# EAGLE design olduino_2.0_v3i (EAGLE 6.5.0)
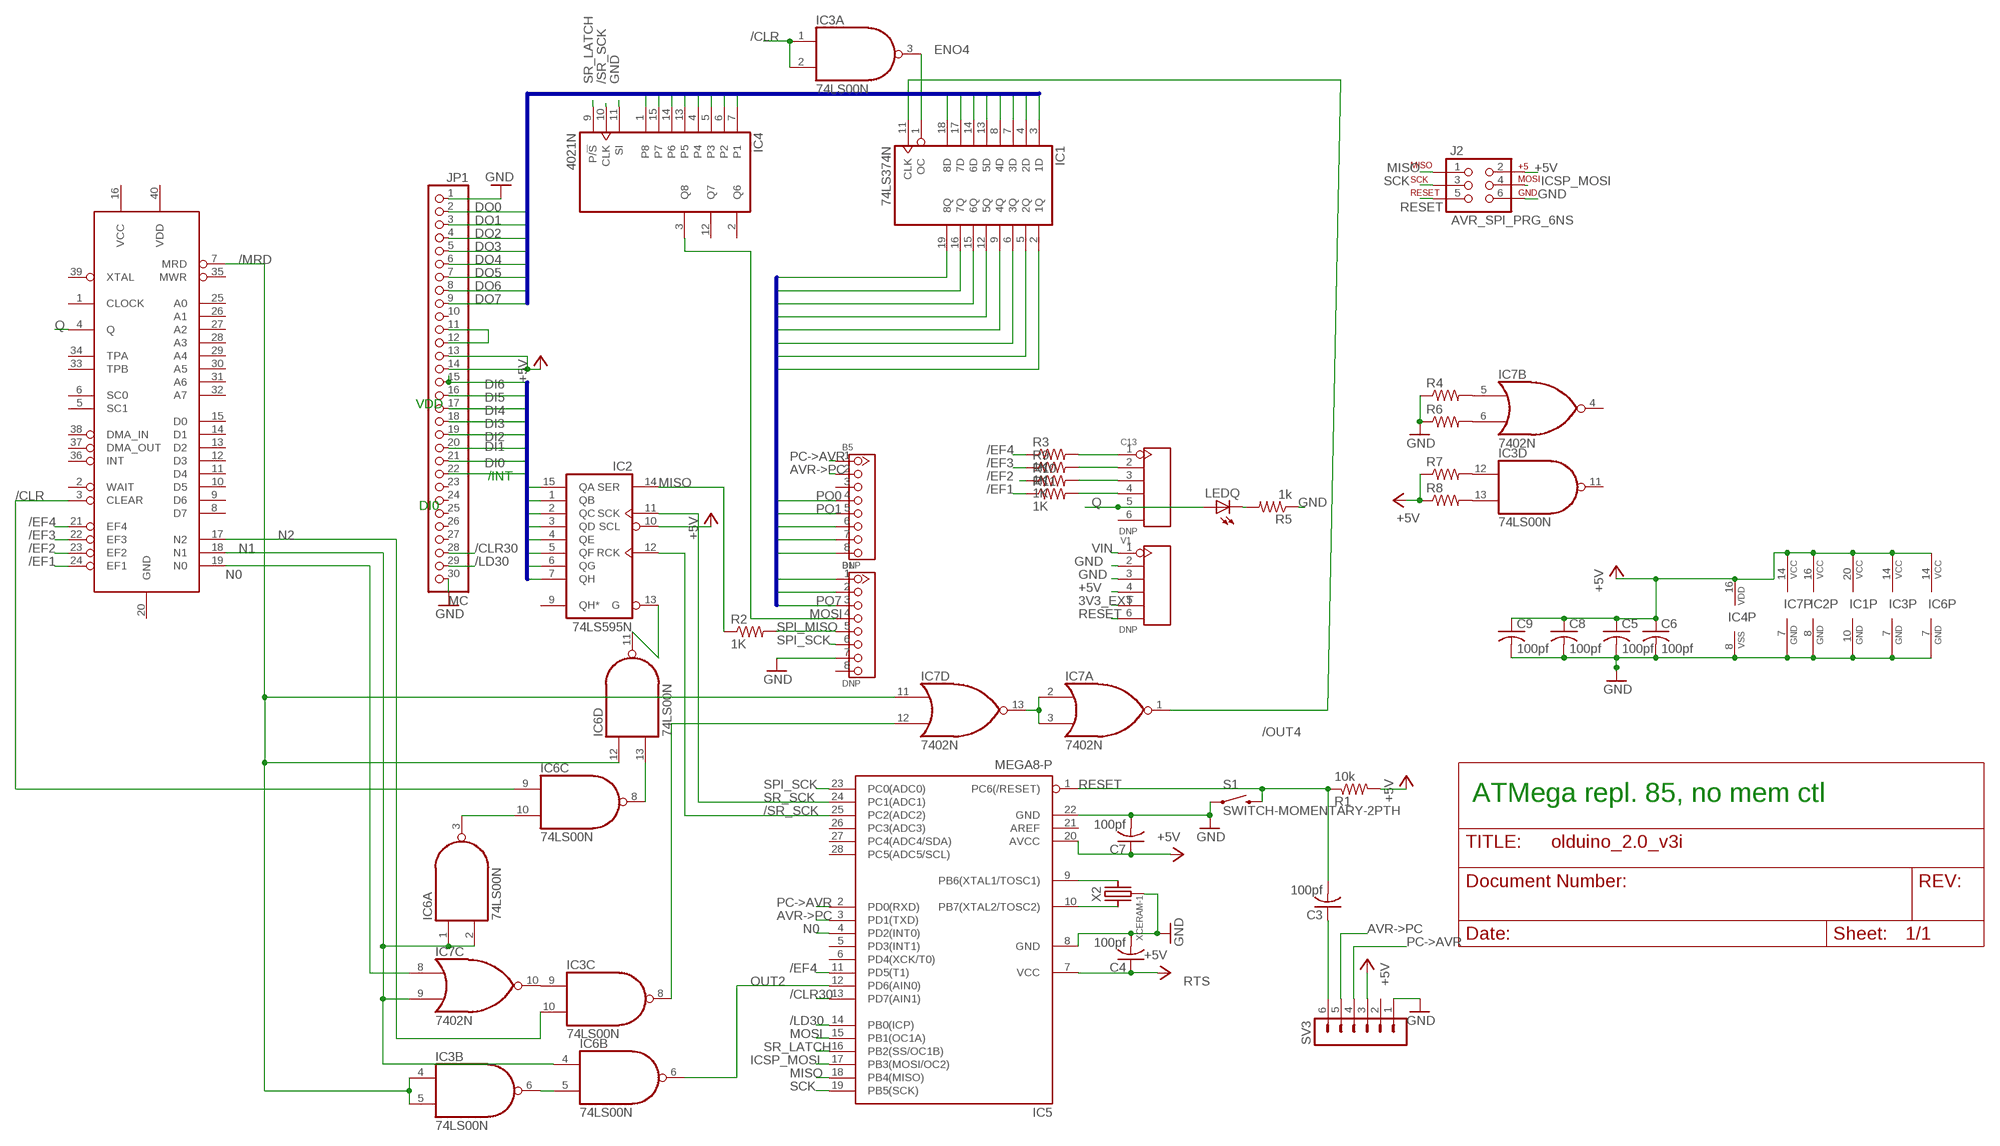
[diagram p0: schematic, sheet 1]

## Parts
B1  DNP  CK_1X8DD  [CK_1X8]
B5  DNP  CK_1X8DD  [CK_1X8]
C3  100pf  C-US025-025X050  [C025-025X050]
C4  100pf  C-US025-025X050  [C025-025X050]
C5  100pf  C-US025-025X050  [C025-025X050]
C6  100pf  C-US025-025X050  [C025-025X050]
C7  100pf  C-US025-025X050  [C025-025X050]
C8  100pf  C-US025-025X050  [C025-025X050]
C9  100pf  C-US025-025X050  [C025-025X050]
C13  DNP  CK_16  [CK_1*6]
IC1  74LS374N  [DIL20]
IC2  74LS595N  [DIL16]
IC3  74LS00N  [DIL14]
IC4  4021N  [DIL16]
IC5  MEGA8-P  [DIL28-3]
IC6  74LS00N  [DIL14]
IC7  7402N  [DIL14]
IC8  CDP1802BCE  CDP1802BCECDP1802BCE  [DIL40]
J2  AVR_SPI_PRG_6NS  [2X3-NS]
JP1  MC  PINHEAD_PINHD-1X30  [PINHEAD_1X30]
LEDQ  LED3MM  [LED3MM]
R1  10k  R-US_0204/2V  [0204V]
R2  1K  R-US_0204/2V  [0204V]
R3  1K  R-US_0204/2V  [0204V]
R4  R-US_0204/2V  [0204V]
R5  1k  R-US_0204/2V  [0204V]
R6  R-US_0204/2V  [0204V]
R7  R-US_0204/2V  [0204V]
R8  R-US_0204/2V  [0204V]
R9  1K  R-US_0204/2V  [0204V]
R10  1K  R-US_0204/2V  [0204V]
R11  1K  R-US_0204/2V  [0204V]
S1  SWITCH-MOMENTARY-2PTH  [TACTILE-PTH]
SV3  MA06-1  [MA06-1]
V1  DNP  CK_16  [CK_1*6]
X2  XCERAM-1  [XTAL-3]

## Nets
3V3_EXT: V1.5
+5V [power]: C4.1 C5.1 C6.1 C7.1 C8.1 C9.1 IC1.20(VCC) IC2.10(SCL) IC2.16(VCC) IC3.14(P:VCC) IC4.16(VDD) IC5.7(VCC) IC5.20(AVCC) IC6.14(P:VCC) IC7.14(P:VCC) J2.2 JP1.13 JP1.14 R1.2 R7.1 R8.1 SV3.3 V1.4
/CLR: IC3.1(A:I0) IC3.2(A:I1) IC6.9(C:I0) IC8.3(CLEAR)
/CLR30: IC5.13(PD7(AIN1)) JP1.28
/EF1: IC8.24(EF1) R11.1
/EF2: IC8.23(EF2) R10.1
/EF3: IC8.22(EF3) R9.1
/EF4: IC5.11(PD5(T1)) IC8.21(EF4) R3.1
/LD30: IC5.14(PB0(ICP)) JP1.29
/MRD: IC3.4(B:I0) IC3.5(B:I1) IC6.12(D:I0) IC7.11(D:I0) IC8.7(MRD)
/OUT4: IC1.11(CLK) IC7.1(A:O)
/SR_SCK: IC2.12(RCK) IC4.10(CLK) IC5.25(PC2(ADC2))
AVR->PC: B5.2 IC5.3(PD1(TXD)) SV3.5
DI0: IC2.15(QA) JP1.22
DI1: IC2.1(QB) JP1.21
DI2: IC2.2(QC) JP1.20
DI3: IC2.3(QD) JP1.19
DI4: IC2.4(QE) JP1.18
DI5: IC2.5(QF) JP1.17
DI6: IC2.6(QG) JP1.16
DI7: IC2.7(QH) JP1.15
DO0: IC1.3(1D) IC4.7(P1) JP1.2
DO1: IC1.4(2D) IC4.6(P2) JP1.3
DO2: IC1.7(3D) IC4.5(P3) JP1.4
DO3: IC1.8(4D) IC4.4 JP1.5
DO4: IC1.13(5D) IC4.13(P5) JP1.6
DO5: IC1.14(6D) IC4.14(P6) JP1.7
DO6: IC1.17(7D) IC4.15(P7) JP1.8
DO7: IC1.18(8D) IC4.1(P8) JP1.9
ENO4: IC1.1(OC) IC3.3(A:O)
GND [GND]: B1.7 C4.2 C5.2 C6.2 C7.2 C8.2 C9.2 IC1.10(GND) IC2.8(GND) IC3.7(P:GND) IC4.8(VSS) IC4.11(SI) IC5.8(GND) IC5.22(GND) IC6.7(P:GND) IC7.7(P:GND) J2.6 JP1.1 JP1.30 R4.1 R5.1 R6.1 S1.1 SV3.1 V1.2 V1.3 X2.P$2(GND)
ICSP_MOSI: IC5.17(PB3(MOSI/OC2)) J2.4
IO4: IC3.8(C:O) IC7.12(D:I1)
MISO: IC2.14(SER) IC5.18(PB4(MISO)) J2.1 R2.1
MOSI: B1.4 IC4.3(Q8) IC5.15(PB1(OC1A))
N0: IC5.4(PD2(INT0)) IC7.8(C:I0) IC8.19(N0)
N1: IC6.1(A:I0) IC6.2(A:I1) IC6.4(B:I0) IC7.9(C:I1) IC8.18(N1)
N2: IC3.10(C:I1) IC8.17(N2)
N$1: IC3.6(B:O) IC6.5(B:I1)
N$2: C13.1 R3.2
N$3: JP1.11 JP1.12
N$4: IC2.13(G) IC6.11(D:O)
N$5: IC7.2(A:I0) IC7.3(A:I1) IC7.13(D:O)
N$6: IC5.10(PB7(XTAL2/TOSC2)) X2.P$1
N$7: IC5.9(PB6(XTAL1/TOSC1)) X2.P$3
N$8: IC6.3(A:O) IC6.10(C:I1)
N$9: IC7.5(B:I0) R4.2
N$10: IC7.6(B:I1) R6.2
N$11: LEDQ.K(C) R5.2
N$12 [power]: IC3.12(D:I0) R7.2
N$13 [power]: IC3.13(D:I1) R8.2
N$14: C13.2 R9.2
N$15: C13.3 R10.2
N$16: C13.4 R11.2
N$55: IC3.9(C:I0) IC7.10(C:O)
N$74: IC6.8(C:O) IC6.13(D:I1)
OUT2: IC5.12(PD6(AIN0)) IC6.6(B:O)
PC->AVR: B5.1 IC5.2(PD0(RXD)) SV3.4
PO0: B5.4 IC1.2(1Q)
PO1: B5.5 IC1.5(2Q)
PO2: B5.6 IC1.6(3Q)
PO3: B5.7 IC1.9(4Q)
PO4: B5.8 IC1.12(5Q)
PO5: B1.1 IC1.15(6Q)
PO6: B1.2 IC1.16(7Q)
PO7: B1.3 IC1.19(8Q)
Q: C13.5 IC8.4(Q) LEDQ.A
RESET: C3.2 IC5.1(PC6(/RESET)) J2.5 R1.1 S1.3 V1.6
RTS: C3.1 SV3.6
SCK: IC5.19(PB5(SCK)) J2.3
SPI_MISO: B1.5 R2.2
SPI_SCK: B1.6 IC5.23(PC0(ADC0))
SR_LATCH: IC4.9(P/!S) IC5.16(PB2(SS/OC1B))
SR_SCK: IC2.11(SCK) IC5.24(PC1(ADC1))
VIN: V1.1
Unconnected: B1.8 B5.3 C13.6 IC2.9(QH*) IC3.11(D:O) IC4.2(Q6) IC4.12(Q7) IC5.5(PD3(INT1)) IC5.6(PD4(XCK/T0)) IC5.21(AREF) IC5.26(PC3(ADC3)) IC5.27(PC4(ADC4/SDA)) IC5.28(PC5(ADC5/SCL)) IC7.4(B:O) IC8.1(CLOCK) IC8.2(WAIT) IC8.5(SC1) IC8.6(SC0) IC8.8(D7) IC8.9(D6) IC8.10(D5) IC8.11(D4) IC8.12(D3) IC8.13(D2) IC8.14(D1) IC8.15(D0) IC8.16(VCC) IC8.20(GND) IC8.25(A0) IC8.26(A1) IC8.27(A2) IC8.28(A3) IC8.29(A4) IC8.30(A5) IC8.31(A6) IC8.32(A7) IC8.33(TPB) IC8.34(TPA) IC8.35(MWR) IC8.36(INT) IC8.37(DMA_OUT) IC8.38(DMA_IN) IC8.39(XTAL) IC8.40(VDD) JP1.10 JP1.23 JP1.24 JP1.25 JP1.26 JP1.27 SV3.2

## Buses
DO[0..7]
DI[0..7]
PO[0..7]

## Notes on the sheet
- VDD
- /INT
- DI0
- ATMega repl. 85, no mem ctl

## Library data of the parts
B1 B5 = CONNECTER:CK_1X8
C3-C9 = rcl:C-US: CAPACITOR, American symbol
C13 V1 = CONNECTER:CK_1*6
IC1 = 74xx-us:74*374: Octal D type transparent LATCH, edge triggered
IC2 = 74xx-us:74*595: 8-bit SHIFT REGISTER, output latch
IC3 IC6 = 74xx-us:74*00: Quad 2-input NAND gate
IC4 = 40xx:4021: 8-bit static SHIFT REGISTER
IC5 = atmel:MEGA8-P: MICROCONTROLLER 8 Kbytes FLASH, 1 kbytes SRAM, 512 bytes EEPROM, USART, 4-channel 10 bit ADC, 2-channel 8 bit ADC Pin compatible with Atmega48, ATMega88, ATMega168 Source: avr.lbr; OC_FARNELL: unknown; OC_NEWARK: unknown
IC7 = 74xx-us:74*02: Quad 2-input NOR gate
IC8 = cdp:CDP1802BCE
J2 = SparkFun-Connectors:AVR_SPI_PRG_6: AVR ISP 6 Pin This is the reduced ISP connector for AVR programming. Common on Arduino. This footprint will take up less PCB space and can be used with a 10-pin to 6-pin adapter such as SKU: BOB-08508
JP1 = olduinov1_ck1:PINHEAD_PINHD-1X30: PIN HEADER
LEDQ = led:LED: LED
R1-R11 = rcl:R-US_: RESISTOR, American symbol
S1 = SparkFun-Electromechanical:SWITCH-MOMENTARY-2: Various NO switches- pushbuttons, reed, etc
SV3 = con-lstb:MA06-1: PIN HEADER; OC_FARNELL: unknown; OC_NEWARK: unknown
X2 = mylib4:XCERAM: Ceramic resonator with built-in caps

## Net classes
0 default: width 0.305 mm, clearance 0.305 mm
1 power: width 0.61 mm, clearance 0.406 mm
2 GND: width 0.61 mm, clearance 0.406 mm

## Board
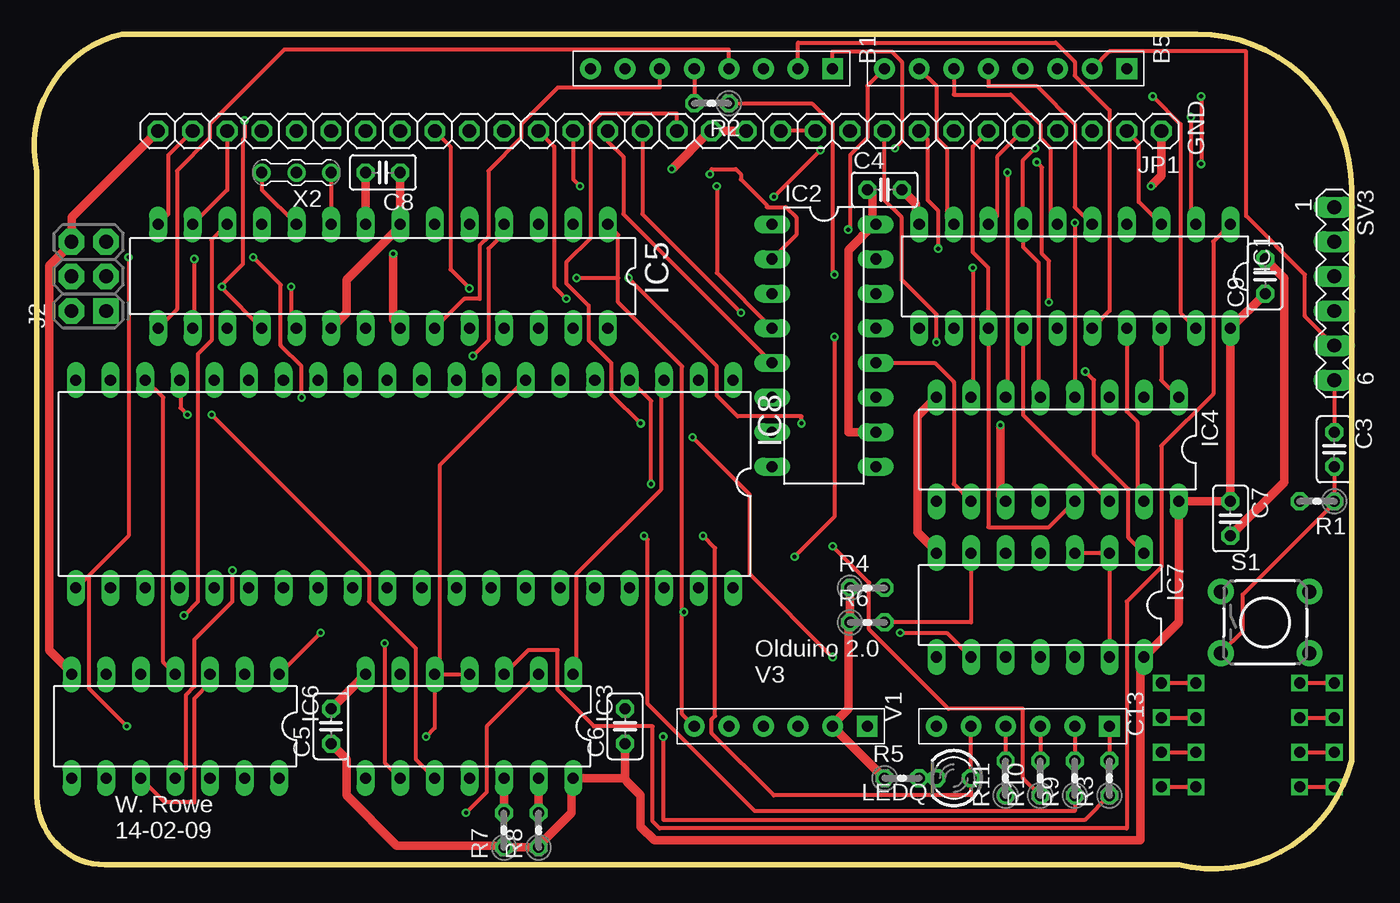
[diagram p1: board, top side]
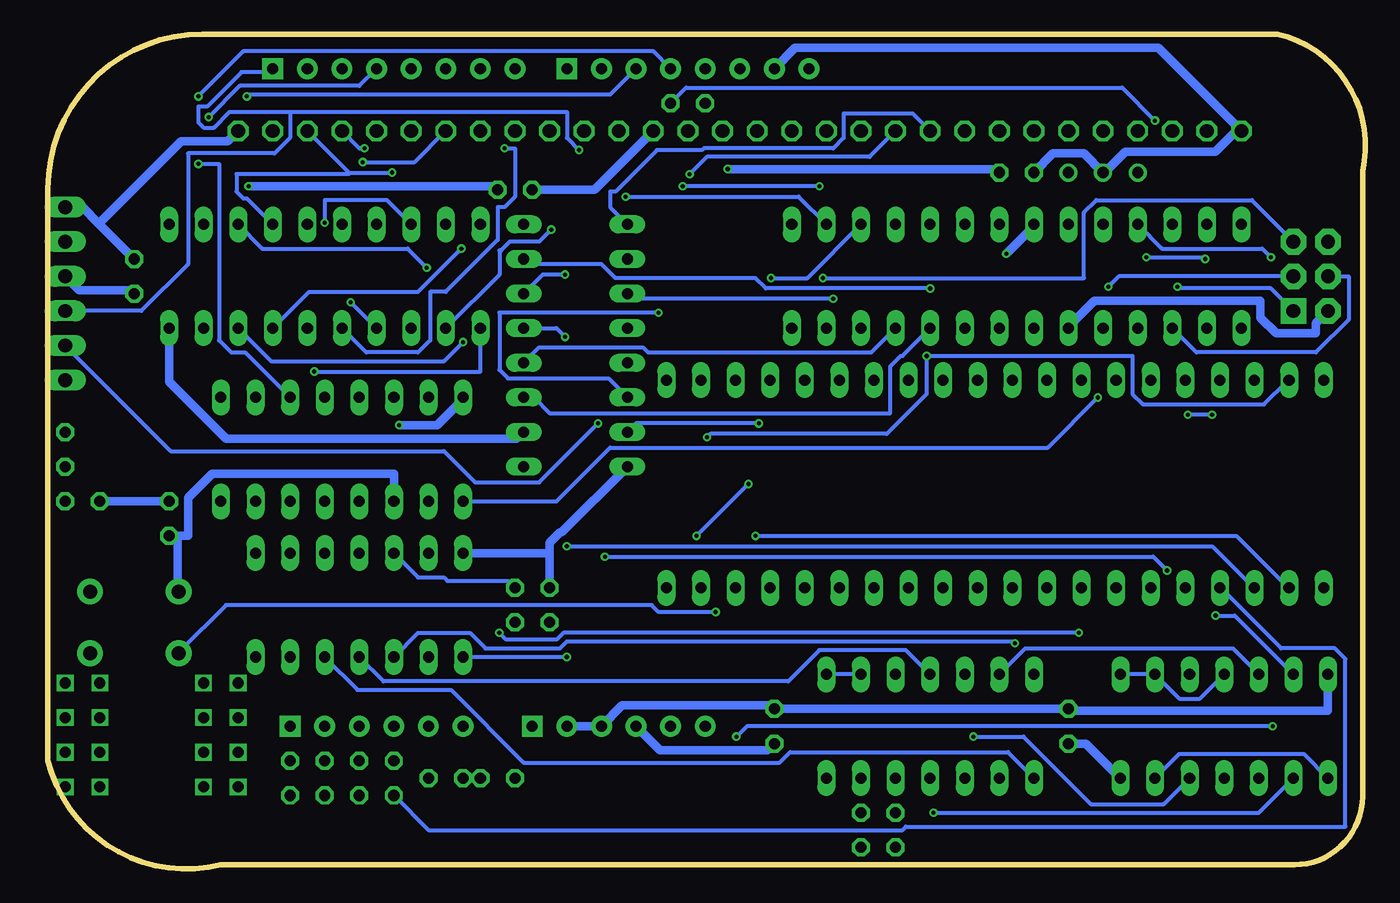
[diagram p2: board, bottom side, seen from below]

Size 96.73 x 61.27 mm. Coordinates in mm from the lower left corner, seen from the top.
Outline: 96.73,49.92 arc90 85.38,61.27 6.48,61.27 arc90 0.21,51.19 0.21,5.31 arc90 5.21,0.31 84.03,0.31 arc90 96.73,7.93 96.73,49.84
Copper layers (1*16): Top 0.035mm / dielectric 1.5mm / Bottom 0.035mm
Design rules "Fusion_eagle_rule_v1.1": minimum track width 6mil, minimum drill 12mil, track to track 6mil, track to pad 6mil, pad to pad 6mil, via to via 6mil, smd to smd 0mil, copper to edge 10mil, drill to drill 10mil, minimum pad ring 10mil, minimum via ring 6mil, stop-mask expansion 2mil, vias tented up to drill 100mil, thermal gap 10mil

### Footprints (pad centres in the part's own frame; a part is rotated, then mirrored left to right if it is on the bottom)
CK_1X8 = drill 0.813 pad 1.524 square: 1 0,8.89 | drill 0.813 pad 1.524: 2 0,6.35; 3 0,3.81; 4 0,1.27; 5 0,-1.27; 6 0,-3.81; 7 0,-6.35; 8 0,-8.89
C025-025X050 = drill 0.813 octagon: 1 -1.27,0; 2 1.27,0
CK_1*6 = drill 0.813 pad 1.524 square: 1 0,6.35 | drill 0.813 pad 1.524: 2 0,3.81; 3 0,1.27; 4 0,-1.27; 5 0,-3.81; 6 0,-6.35
DIL20 = drill 0.813 long: 1 -11.43,-3.81; 2 -8.89,-3.81; 3 -6.35,-3.81; 4 -3.81,-3.81; 5 -1.27,-3.81; 6 1.27,-3.81; 7 3.81,-3.81; 8 6.35,-3.81; 9 8.89,-3.81; 10 11.43,-3.81; 11 11.43,3.81; 12 8.89,3.81; 13 6.35,3.81; 14 3.81,3.81; 15 1.27,3.81; 16 -1.27,3.81; 17 -3.81,3.81; 18 -6.35,3.81; 19 -8.89,3.81; 20 -11.43,3.81
DIL16 = drill 0.813 long: 1 -8.89,-3.81; 2 -6.35,-3.81; 3 -3.81,-3.81; 4 -1.27,-3.81; 5 1.27,-3.81; 6 3.81,-3.81; 7 6.35,-3.81; 8 8.89,-3.81; 9 8.89,3.81; 10 6.35,3.81; 11 3.81,3.81; 12 1.27,3.81; 13 -1.27,3.81; 14 -3.81,3.81; 15 -6.35,3.81; 16 -8.89,3.81
DIL14 = drill 0.813 long: 1 -7.62,-3.81; 2 -5.08,-3.81; 3 -2.54,-3.81; 4 0,-3.81; 5 2.54,-3.81; 6 5.08,-3.81; 7 7.62,-3.81; 8 7.62,3.81; 9 5.08,3.81; 10 2.54,3.81; 11 0,3.81; 12 -2.54,3.81; 13 -5.08,3.81; 14 -7.62,3.81
DIL28-3 = drill 0.813 long: 1 -16.51,-3.81; 2 -13.97,-3.81; 3 -11.43,-3.81; 4 -8.89,-3.81; 5 -6.35,-3.81; 6 -3.81,-3.81; 7 -1.27,-3.81; 8 1.27,-3.81; 9 3.81,-3.81; 10 6.35,-3.81; 11 8.89,-3.81; 12 11.43,-3.81; 13 13.97,-3.81; 14 16.51,-3.81; 15 16.51,3.81; 16 13.97,3.81; 17 11.43,3.81; 18 8.89,3.81; 19 6.35,3.81; 20 3.81,3.81; 21 1.27,3.81; 22 -1.27,3.81; 23 -3.81,3.81; 24 -6.35,3.81; 25 -8.89,3.81; 26 -11.43,3.81; 27 -13.97,3.81; 28 -16.51,3.81
DIL40 = drill 0.813 long: 1 -24.13,-7.62; 2 -21.59,-7.62; 3 -19.05,-7.62; 4 -16.51,-7.62; 5 -13.97,-7.62; 6 -11.43,-7.62; 7 -8.89,-7.62; 8 -6.35,-7.62; 9 -3.81,-7.62; 10 -1.27,-7.62; 11 1.27,-7.62; 12 3.81,-7.62; 13 6.35,-7.62; 14 8.89,-7.62; 15 11.43,-7.62; 16 13.97,-7.62; 17 16.51,-7.62; 18 19.05,-7.62; 19 21.59,-7.62; 20 24.13,-7.62; 21 24.13,7.62; 22 21.59,7.62; 23 19.05,7.62; 24 16.51,7.62; 25 13.97,7.62; 26 11.43,7.62; 27 8.89,7.62; 28 6.35,7.62; 29 3.81,7.62; 30 1.27,7.62; 31 -1.27,7.62; 32 -3.81,7.62; 33 -6.35,7.62; 34 -8.89,7.62; 35 -11.43,7.62; 36 -13.97,7.62; 37 -16.51,7.62; 38 -19.05,7.62; 39 -21.59,7.62; 40 -24.13,7.62
2X3-NS = drill 1.016 pad 1.88 square: 1 -2.54,-1.27 | drill 1.016 pad 1.88 octagon: 2 -2.54,1.27; 3 0,-1.27; 4 0,1.27; 5 2.54,-1.27; 6 2.54,1.27
PINHEAD_1X30 = drill 1.016 octagon: 1 -36.83,0; 2 -34.29,0; 3 -31.75,0; 4 -29.21,0; 5 -26.67,0; 6 -24.13,0; 7 -21.59,0; 8 -19.05,0; 9 -16.51,0; 10 -13.97,0; 11 -11.43,0; 12 -8.89,0; 13 -6.35,0; 14 -3.81,0; 15 -1.27,0; 16 1.27,0; 17 3.81,0; 18 6.35,0; 19 8.89,0; 20 11.43,0; 21 13.97,0; 22 16.51,0; 23 19.05,0; 24 21.59,0; 25 24.13,0; 26 26.67,0; 27 29.21,0; 28 31.75,0; 29 34.29,0; 30 36.83,0
LED3MM = drill 0.813 octagon: A -1.27,0; K 1.27,0
0204V = drill 0.813 octagon: 1 -1.27,0; 2 1.27,0
TACTILE-PTH = drill 1.016 pad 1.88: 1 -3.251,2.261; 2 3.251,2.261; 3 -3.251,-2.261; 4 3.251,-2.261
MA06-1 = drill 1.016 long: 1 -6.35,0; 2 -3.81,0; 3 -1.27,0; 4 1.27,0; 5 3.81,0; 6 6.35,0
XTAL-3 = drill 0.813: P$1 0,2.54; P$2 0,0; P$3 0,-2.54

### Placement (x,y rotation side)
B1  49.74,58.73 270 top
B5  71.33,58.73 270 top
C3  95.46,30.79 270 top
C4  62.44,49.84 0 top
C5  21.8,10.47 90 top
C6  43.39,10.47 90 top
C7  87.84,25.71 270 top
C8  25.61,51.11 180 top
C9  90.38,43.49 90 top
C13  72.6,10.47 270 top
IC1  76.41,43.49 180 top
IC2  58,38.41 270 top
IC3  31.96,10.47 180 top
IC4  75.14,30.79 180 top
IC5  25.61,43.49 180 top
IC6  10.37,10.47 180 top
IC7  73.87,19.36 180 top
IC8  27.2,28.25 180 top
J2  4.02,43.49 90 top
JP1  45.93,54.16 180 top
LEDQ  67.52,6.66 180 top
R1  94.19,26.98 180 top
R2  49.74,56.19 180 top
R3  78.95,6.66 90 top
R4  61.17,20.63 0 top
R5  63.71,6.66 0 top
R6  61.17,18.09 0 top
R7  34.5,2.85 90 top
R8  37.04,2.85 90 top
R9  76.41,6.66 90 top
R10  73.87,6.66 90 top
R11  71.33,6.66 90 top
S1  90.38,18.09 0 top
SV3  95.46,42.22 270 top
V1  54.82,10.47 270 top
X2  19.26,51.11 90 top

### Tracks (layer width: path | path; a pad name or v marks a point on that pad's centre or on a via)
+5V  (via drill 0.3)
  Top 0.61: 43.39,6.66 IC3.14 39.45,6.4 39.45,4.12 37.17,1.83 R8.1 R7.1 34.25,1.7 26.63,1.7 22.94,5.39 22.94,8.05 C5.1 | C6.1 43.39,6.66 | IC5.20 22.94,40.82 22.94,43.23 26.88,47.17 IC5.7 C8.1 | JP1.13 JP1.14 49.49,54.03 v46.82,51.36 | IC2.10 59.77,32.06 59.77,45.39 61.68,47.3 IC2.16 61.55,47.55 61.55,49.46 C4.1 | C9.1 IC1.20 C7.1 IC4.16 84.03,18.09 IC7.14 81.24,15.42 81.24,2.09 45.55,2.09 44.53,3.1 44.53,5.39 43.52,6.4 43.39,6.66
  Bottom 0.61: IC6.14 20.53,9.2 C5.1 | V1.4 51.77,8.69 43.9,8.69 C6.1 | J2.2 3.64,40.06 3.64,39.3 6.56,39.3 7.7,40.44 7.7,41.71 19.9,41.71 21.8,39.8 IC5.20 | JP1.13 56.6,49.84 C4.1 | SV3.3 94.44,42.47 90.63,42.47 C9.1 | C7.1 R1.2 | IC2.10 62.31,31.55 83.65,31.55 87.84,35.74 IC1.20 | C8.1 27.13,51.36 v46.82,51.36
/CLR  (via drill 0.3)
  Top 0.305: v31.71,4.12 33.23,5.64 33.23,10.47 IC3.2 | IC3.1 39.83,14.53 39.83,21.64 46.06,27.87 46.06,35.74 46.18,35.87 IC8.3
  Bottom 0.305: IC6.9 7.83,4.12 v31.71,4.12 | IC3.2 IC3.1
/CLR30
  Top 0.305: IC5.13 14.18,49.84 JP1.28
/EF1
  Bottom 0.305: R11.1 68.79,2.85 33.99,2.85 33.74,3.1 1.48,3.1 1.48,15.42 2.24,16.18 6.18,16.18 10.62,20.63 IC8.24
/EF2  (via drill 0.3)
  Top 0.305: v58.63,23.68 61.3,21.01 61.3,17.58 67.14,11.74 72.6,11.74 72.6,6.66 R10.1
  Bottom 0.305: v58.63,23.68 11.26,23.68 8.21,20.63 IC8.23
/EF3  (via drill 0.3)
  Top 0.305: v44.79,24.44 45.04,24.18 45.04,12.12 52.92,4.24 76.41,4.24 R9.1
  Bottom 0.305: v44.79,24.44 9.48,24.44 5.67,20.63 IC8.22
/EF4  (via drill 0.3)
  Top 0.305: 3.96,21.45 6.94,24.44 v6.94,44.88 | 3.96,21.45 3.13,20.63 IC8.21 | R3.1 77.17,3.61 46.18,3.61 v46.18,9.71 | v6.81,10.47 4.02,13.26 4.02,21.39 3.96,21.45
  Bottom 0.305: v6.94,44.88 7.58,45.52 14.94,45.52 IC5.11 | v46.18,9.71 45.42,10.47 v6.81,10.47
/LD30
  Top 0.305: IC5.14 9.86,48.06 9.86,52.38 JP1.29
/MRD  (via drill 0.3)
  Top 0.305: v28.79,9.71 29.42,10.34 IC3.5 | IC3.5 IC3.4 | IC8.7 36.02,35.87 29.8,29.64 29.8,14.4 IC3.5
  Bottom 0.305: IC6.12 14.82,4.75 20.15,4.75 25.1,9.71 v28.79,9.71 | IC7.11 72.09,13.77 42.37,13.77 40.09,16.06 33.74,16.06 IC3.4
/OUT4  (via drill 0.3)
  Top 0.305: v77.17,36.5 77.81,35.87 77.81,30.41 80.35,27.87 80.35,24.31 IC7.1
  Bottom 0.305: IC1.11 64.98,36.5 v77.17,36.5
/SR_SCK
  Top 0.305: IC4.10 67.52,28.25 67.52,35.74 66.12,37.14 IC2.12
  Bottom 0.305: IC5.25 36.28,37.9 52.66,37.9 53.04,38.28 60.66,38.28 IC2.12
AVR->PC  (via drill 0.3)
  Top 0.305: v43.64,43.36 50.12,36.88 50.12,34.72 51.65,33.2 56.34,33.2 v56.34,32.69 | B5.2 78.95,60 88.98,60 88.98,47.93 93.3,43.61 93.3,40.57 SV3.5
  Bottom 0.305: IC5.3 40.98,43.36 v43.64,43.36 | v56.34,32.69 60.66,28.37 65.36,28.37 67.65,30.66 87.71,30.66 SV3.5
DI0  (via drill 0.3)
  Top 0.305: v31.96,42.6 30.56,44 30.56,53.01 JP1.22
  Bottom 0.305: IC2.15 61.42,44.38 56.09,44.38 55.07,43.36 44.79,43.36 44.03,42.6 v31.96,42.6
DI1
  Bottom 0.305: IC2.1 55.46,48.57 55.46,49.71 55.07,49.71 52.03,52.76 48.72,52.76 48.6,52.89 39.07,52.89 38.31,53.65 38.31,55.43 33.23,55.43 JP1.21
DI2  (via drill 0.3)
  Top 0.305: IC2.2 55.96,46.54 55.96,47.81 55.2,48.57 53.8,48.57 53.8,48.69 51.9,50.6 51.9,50.98 51.52,51.36 49.74,51.36 49.74,51.11 v49.61,50.98
  Bottom 0.305: v49.61,50.98 48.34,52.25 36.41,52.25 JP1.20
DI3  (via drill 0.3)
  Top 0.305: v39.07,41.84 38.18,42.73 38.18,53.01 JP1.19
  Bottom 0.305: IC2.3 53.8,41.84 v39.07,41.84
DI4  (via drill 0.3)
  Top 0.305: IC2.4 50.12,43.74 v50.12,50.09 | v40.09,50.09 39.58,50.6 JP1.18
  Bottom 0.305: v40.09,50.09 v50.12,50.09
DI5
  Top 0.305: IC2.5 43.26,48.06 43.26,52.25 42.12,53.39 JP1.17
DI6  (via drill 0.3)
  Top 0.305: v51.9,40.82 44.66,48.06 JP1.16
  Bottom 0.305: IC2.6 55.58,35.99 62.95,35.99 63.58,36.63 63.58,40.82 v51.9,40.82
DI7  (via drill 0.3)
  Top 0.305: v44.53,32.69 42.37,34.85 42.37,37.14 40.72,38.79 40.72,41.33 39.07,42.98 39.07,44.5 40.85,46.28 40.85,54.66 41.61,55.43 47.2,55.43 JP1.15
  Bottom 0.305: IC2.7 53.55,32.69 v44.53,32.69
DO0  (via drill 0.3)
  Top 0.305: IC4.7 68.92,34.72 v68.92,44.12 | JP1.2 81.11,53.27 81.11,48.95 IC1.3
  Bottom 0.305: v68.92,44.12 70.31,45.52 80.98,45.52 IC1.3
DO1  (via drill 0.3)
  Top 0.305: IC4.6 71.46,34.72 v71.46,51.11
  Bottom 0.305: 74.63,51.11 v71.46,51.11 | JP1.3 74.63,51.11 | IC1.4 82.13,49.2 82.38,49.2 82.89,49.71 82.89,50.98 74.63,50.98 74.63,51.11
DO2  (via drill 0.3)
  Top 0.305: IC4.5 73.74,34.72 73.74,44.5 72.6,45.65 IC1.7 72.6,52 v73.49,52.89
  Bottom 0.305: JP1.4 73.87,52.89 v73.49,52.89
DO3  (via drill 0.3)
  Top 0.305: IC1.8 70.7,47.93 70.7,52.25 JP1.5 | v76.41,47.42 IC4.4
  Bottom 0.305: v76.41,47.42 76.41,49.08 71.84,49.08 IC1.8
DO4
  Top 0.305: IC4.13 74.51,25.07 70.06,25.07 IC1.13 70.06,44.12 68.92,45.27 68.92,53.01 JP1.6
DO5  (via drill 0.3)
  Top 0.305: IC4.14 72.6,33.33 IC1.14 | v73.62,51.87 74,51.49 74,45.14 74.51,44.63 v74.51,41.58
  Bottom 0.305: JP1.7 69.81,51.87 v73.62,51.87 | IC1.14 v74.51,41.58
DO6  (via drill 0.3)
  Top 0.305: IC4.15 80.98,27.49 80.98,32.82 80.22,33.58 IC1.17 | JP1.8 65.62,53.52 65.62,49.08 66.38,48.31 v66.38,45.52
  Bottom 0.305: v66.38,45.52 69.55,42.34 77.55,42.34 IC1.17
DO7  (via drill 0.3)
  Top 0.305: IC4.1 82.76,35.87 IC1.18 | JP1.9 62.44,49.08 63.71,47.81 63.71,43.23 66.25,40.69 v66.25,38.66
  Bottom 0.305: v66.25,38.66 67.65,37.26 80.35,37.26 IC1.18
ENO4
  Top 0.305: IC3.3 36.28,16.06 38.44,16.06 38.44,13.13 41.1,10.47 45.42,10.47 45.42,3.48 45.93,2.97 80.22,2.97 80.22,19.61 82.76,22.15 82.76,31.04 86.57,34.85 86.57,46.03 IC1.1
GND  (via drill 0.3)
  Top 0.61: C4.2 64.73,48.82 64.73,47.55 IC1.10 | v82,50.09 82.76,50.85 JP1.1 | C7.2 91.78,28.37 91.78,43.36 C9.2 | C8.2 IC5.8 | v26.37,45.14 26.37,40.31 26.75,39.93 IC5.22 | JP1.30 2.75,47.81 J2.6 2.62,45.77 1.1,44.25 1.1,16.06 2.62,14.53 IC6.7 | IC3.7 C5.2 | R5.1 V1.2 58.76,10.72 59.77,11.74 59.77,17.83 R6.1 R4.1 | IC4.8 64.85,33.2 64.85,24.69 66.12,23.42 IC7.7 | IC4.11 70.95,27.36 v70.95,32.57
  Bottom 0.61: IC4.11 71.33,29.01 84.67,29.01 86.44,27.23 86.44,24.44 C7.2 87.21,24.18 87.21,20.37 S1.1 | 92.98,47.36 94.19,48.57 SV3.1 | 92.98,47.36 C9.2 | JP1.1 83.52,53.39 86.95,53.39 92.98,47.36 | C4.2 63.96,50.09 v82,50.09 | v26.37,45.14 24.34,47.17 IC5.8 | C8.2 22.94,52.5 20.66,52.5 X2.P$2 19.01,51.23 17.61,52.63 11.01,52.63 9.48,54.16 JP1.30 15.2,60.25 41.87,60.25 B1.7 | IC6.7 2.75,11.61 21.67,11.61 C5.2 C6.2 43.64,11.99 54.57,11.99 V1.3 V1.2 | IC2.8 59.01,24.69 59.14,24.69 59.9,23.93 59.9,23.17 | R4.1 59.9,23.17 | 59.9,23.17 IC7.7 | v70.95,32.57 68.16,32.57 66.25,34.47 IC4.8
ICSP_MOSI
  Bottom 0.305: IC5.17 12.4,37.9 3.64,37.9 1.23,40.31 1.23,43.49 J2.4
IO4
  Bottom 0.305: IC3.8 26.25,8.56 42.25,8.56 43.01,7.8 61.81,7.8 67.14,13.13 74,13.13 IC7.12
MISO  (via drill 0.3)
  Top 0.305: IC5.18 13.8,42.6 v13.8,42.73 13.8,42.85 15.32,44.38 15.32,53.52 15.45,53.65 v15.45,54.92 | v58.76,43.61 58.63,43.74 58.63,54.66 57.11,56.19 R2.1
  Bottom 0.305: v13.8,42.73 13.67,42.6 6.94,42.6 J2.1 | IC2.14 60.41,43.61 v58.76,43.61 | v15.45,54.92 17.86,57.33 49.87,57.33 R2.1
MOSI  (via drill 0.3)
  Top 0.305: IC5.15 10.5,41.07 10.5,51.23 12.91,53.65 12.91,54.66 18.37,60.12 51.01,60.12 B1.4 | v85.68,56.7 v85.68,51.74
  Bottom 0.305: IC4.3 82.25,37.9 83.27,37.9 84.16,38.79 84.16,51.74 v85.68,51.74 | v85.68,56.7 82.38,60 52.28,60 B1.4
N0  (via drill 0.3)
  Top 0.305: v32.21,37.65 33.36,38.79 33.36,45.52 34.5,46.66 IC5.4 | v58.63,15.55 52.53,21.64 52.53,27.49 v48.34,31.68
  Bottom 0.305: IC8.19 5.67,35.87 7.45,34.09 16.34,34.09 17.1,34.85 17.1,37.65 v32.21,37.65 32.21,34.85 35.14,31.93 48.09,31.93 v48.34,31.68 | v58.63,15.55 IC7.8
N1  (via drill 0.3)
  Top 0.305: IC6.4 9.48,15.17 9.48,34.6 8.21,35.87 IC8.18 | IC7.9 67.01,17.33 v63.58,17.33 | IC6.1 v21.04,17.33
  Bottom 0.305: IC6.4 12.15,12.5 13.67,12.5 IC6.2 IC6.1 | v63.58,17.33 63.08,16.82 59.39,16.82 58.88,17.33 v21.04,17.33
N2  (via drill 0.3)
  Top 0.305: IC3.10 28.02,8.05 28.02,16.18 24.59,19.61 24.59,21.77 v13.04,33.33 | v11.26,33.33 10.75,33.84 10.75,35.87 IC8.17
  Bottom 0.305: v11.26,33.33 v13.04,33.33
N$1
  Bottom 0.305: IC6.5 9.74,16.18 24.98,16.18 IC3.6
N$2
  Top 0.305: C13.1 R3.2
N$3
  Top 0.305: JP1.11 JP1.12
N$4  (via drill 0.3)
  Top 0.305: IC6.11 11.13,7.42 11.13,12.75 11.77,13.39 11.77,16.82 14.56,19.61 v14.56,21.9 | v55.84,22.91 58.76,25.83 v58.76,39.04
  Bottom 0.305: v14.56,21.9 15.58,22.91 v55.84,22.91 | v58.76,39.04 59.39,39.68 IC2.13
N$5
  Top 0.305: IC7.3 IC7.2 IC7.13
N$6
  Top 0.305: IC5.10 16.72,49.84 X2.P$1
N$7
  Top 0.305: X2.P$3 IC5.9
N$8
  Top 0.305: IC6.10 9.61,4.88 11.77,4.88 11.77,12.5 12.91,13.64 IC6.3
N$9
  Bottom 0.305: R4.2 62.95,21.14 67.39,21.14 67.65,21.39 69.55,21.39 IC7.5
N$10
  Top 0.305: R6.2 68.79,18.09 IC7.6
N$11
  Top 0.305: LEDQ.K R5.2
N$12
  Top 0.61: IC3.12 R7.2
N$13
  Top 0.61: IC3.13 R8.2
N$14
  Top 0.305: C13.2 R9.2
N$15
  Top 0.305: C13.3 R10.2
N$16
  Top 0.305: C13.4 R11.2
N$17  (via drill 0.81)
  Top 0.305: v92.92,11.1 v95.46,11.1
N$18  (via drill 0.81)
  Top 0.305: v92.92,8.56 v95.46,8.56
N$19  (via drill 0.81)
  Top 0.305: v92.92,6.02 v95.46,6.02
N$20  (via drill 0.81)
  Top 0.305: v82.76,11.1 v85.3,11.1
N$21  (via drill 0.81)
  Top 0.305: v82.76,8.56 v85.3,8.56
N$22  (via drill 0.81)
  Top 0.305: v92.92,13.64 v95.46,13.64
N$23  (via drill 0.81)
  Top 0.305: v82.76,6.02 v85.3,6.02
N$24  (via drill 0.81)
  Top 0.305: v82.76,13.64 v85.3,13.64
N$55  (via drill 0.3)
  Top 0.305: IC3.9 25.74,7.8 v25.74,16.56
  Bottom 0.305: v25.74,16.56 25.86,16.69 58.63,16.69 59.14,16.18 64.6,16.18 65.74,17.33 69.55,17.33 IC7.10
N$74
  Bottom 0.305: IC6.8 4.53,8.44 13.67,8.44 IC6.13
OUT2  (via drill 0.3)
  Top 0.305: v11.01,18.6 12.02,19.61 12.02,37.77 13.04,38.79 13.04,46.15 IC5.12
  Bottom 0.305: IC6.6 9.61,18.6 v11.01,18.6
PC->AVR  (via drill 0.3)
  Top 0.305: v57.74,52.76 v54.31,49.33
  Bottom 0.305: IC5.2 41.61,49.33 v54.31,49.33 | v57.74,52.76 58.63,53.65 58.63,55.55 78.95,55.55 | 78.95,55.55 83.4,55.55 84.54,54.41 85.3,54.41 85.68,54.79 85.68,55.93 85.05,55.93 82.51,58.47 80.47,58.47 B5.1 | SV3.4 89.87,40.95 86.44,44.38 86.44,52.5 80.09,52.5 78.95,53.65 78.95,55.55
PO0  (via drill 0.3)
  Top 0.305: IC1.2 84.92,47.68 v84.92,55.17
  Bottom 0.305: v84.92,55.17 82.63,57.46 73.87,57.46 B5.4
PO1
  Top 0.305: IC1.5 76.41,48.57 76.41,54.66 73.62,57.46 70.06,57.46 B5.5
PO2
  Top 0.305: IC1.6 74.63,47.81 74.63,52.89 73.87,53.65 73.87,54.66 71.71,56.82 67.52,56.82 B5.6
PO3
  Top 0.305: IC1.9 67.01,47.81 67.01,52.89 66.25,53.65 66.25,57.46 B5.7
PO4  (via drill 0.3)
  Top 0.305: v59.77,46.92 59.9,47.04 59.9,52.38 61.17,53.65 61.17,57.46 B5.8
  Bottom 0.305: IC1.12 63.58,43.61 63.58,45.39 63.46,45.39 62.82,46.03 60.66,46.03 v59.77,46.92
PO5  (via drill 0.3)
  Top 0.305: v63.2,52.89 63.71,53.39 63.71,59.24 62.95,60 58.63,60 B1.1
  Bottom 0.305: IC1.15 73.36,37.9 69.55,37.9 68.66,38.79 68.66,42.34 67.52,42.34 63.71,46.15 63.71,48.57 63.2,48.57 62.44,49.33 62.44,52.89 v63.2,52.89
PO6
  Top 0.305: IC1.16 78.95,40.95 78.95,55.68 76.41,58.22 76.41,59.24 75.01,60.63 56.09,60.63 B1.2
PO7  (via drill 0.3)
  Top 0.305: IC1.19 84.16,40.82 84.16,54.66 v82.13,56.7
  Bottom 0.305: v82.13,56.7 82,56.82 55.46,56.82 B1.3
Q  (via drill 0.3)
  Top 0.305: v45.3,28.25 45.3,34.34 43.77,35.87 IC8.4 | v49.11,24.44 49.99,23.55 49.99,11.23 49.74,10.98 49.74,9.96 54.31,5.39 68.79,5.39 LEDQ.A C13.5
  Bottom 0.305: v49.11,24.44 v45.3,28.25
RESET  (via drill 0.3)
  Top 0.305: C3.2 R1.1 95.46,26.85 88.73,20.12 88.73,17.45 87.21,15.93 S1.3 | IC5.1 42.88,46.54 42.88,43.36 | 42.88,43.36 42.88,41.58 47.58,36.88 47.58,18.85 | 47.58,18.85 47.58,11.36 V1.6 | 42.88,43.36 v39.83,43.36 | v47.71,18.85 47.58,18.85
  Bottom 0.305: J2.5 8.34,49.08 19.77,49.08 20.66,48.19 20.66,43.36 v39.83,43.36 | v47.71,18.85 51.9,18.85 52.41,19.36 83.65,19.36 87.08,15.93 S1.3
RTS
  Top 0.305: SV3.6 C3.1
SCK  (via drill 0.3)
  Top 0.305: IC5.19 18.88,40.06 v18.88,42.73
  Bottom 0.305: v18.88,42.73 18.12,43.49 J2.3
SPI_MISO
  Top 0.305: B1.5 R2.2
SPI_SCK
  Top 0.305: IC5.23 31.58,41.84 32.72,41.84 32.72,45.77 33.36,46.41 33.36,51.23 35.77,53.65 35.77,54.66 38.44,57.33 45.93,57.33 B1.6
SR_LATCH  (via drill 0.3)
  Top 0.305: IC5.16 11.77,39.8 v11.77,44.76 | v16.09,44.88 18.12,42.85 18.12,38.41 19.64,36.88 v19.64,34.6
  Bottom 0.305: v11.77,44.76 11.89,44.88 v16.09,44.88 | v19.64,34.6 23.32,30.91 55.46,30.91 59.39,26.98 IC4.9
SR_SCK
  Bottom 0.305: IC5.24 33.99,37.65 34.12,37.65 34.88,36.88 34.88,33.45 59.9,33.45 61.04,34.6 IC2.11

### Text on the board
_tsilk: GND | Olduino 2.0 / V3 | W. Rowe / 14-02-09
